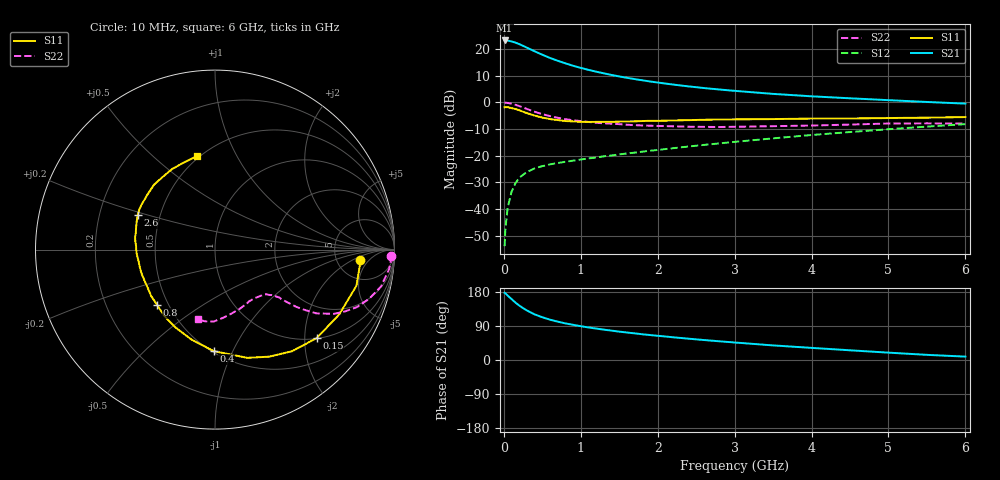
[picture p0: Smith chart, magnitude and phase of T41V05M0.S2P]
! Infineon Technologies  Discrete & RF Semiconductors
! BFR182T
! Si NPN RF Bipolar Junction Transistor in SC75
! VCE = 1 V  IC = 5 mA
! Common Emitter S-Parameters:  October  1999
# GHz  S  MA  R  50
!  f  S11  S21  S12  S22
! GHz  MAG  ANG  MAG  ANG  MAG  ANG  MAG  ANG
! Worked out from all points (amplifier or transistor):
!   36 points, 10 MHz to 6 GHz, reference 50 ohm
!   highest |S21| = 23.2 dB at 10 MHz (marker M1)
!   |S21| within 3 dB of that: start of sweep to 321.7 MHz
!   unconditionally stable (mu >= 1): 1.274 GHz to 4.316 GHz
!   at 250 MHz: K = 0.30, MSG = 24.2 dB, |S12| = -27.2 dB
!   at 1.4 GHz: K = 1.04, MAG = 13.8 dB, |S12| = -19.9 dB
!   at 6 GHz: K = 0.89, MSG = 3.9 dB, |S12| = -8.2 dB
!   S11 on the Smith chart (normalised r, x): 10 MHz: 8.54, -2.78; 150 MHz: 1.01, -2.29; 400 MHz: 0.51, -0.85; 800 MHz: 0.43, -0.34; 2.6 GHz: 0.37, +0.18; 6 GHz: 0.49, +0.70
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0.01  0.8087 -4.0  14.53 177.3  0.002 84.8  0.9805 -2.0
0.02  0.8136 -4.4  14.46 176.3  0.0042 92.8  0.9845 -2.6
0.05  0.8134 -14.3  14.46 170.0  0.0106 87.4  0.9762 -6.4
0.1  0.7809 -27.5  13.93 160.8  0.0209 77.8  0.9478 -12.5
0.15  0.7512 -41.0  13.24 151.6  0.0304 70.2  0.9016 -17.7
0.2  0.7107 -52.8  12.41 143.8  0.0382 65.7  0.8528 -22.1
0.25  0.6688 -63.1  11.51 136.9  0.0439 60.3  0.7997 -25.6
0.3  0.6293 -73.4  10.64 130.7  0.0493 58.3  0.7527 -28.4
0.4  0.5653 -90.8  9.101 120.4  0.0577 53.1  0.6666 -32.2
0.5  0.5179 -104.7  7.839 112.8  0.0636 50.7  0.6024 -33.9
0.6  0.4865 -116.9  6.826 106.4  0.0686 49.8  0.5527 -35.2
0.7  0.4657 -127.3  6.044 101.2  0.0727 49.3  0.5144 -35.8
0.8  0.4465 -136.2  5.409 96.6  0.0767 49.3  0.4848 -36.3
1.1  0.4292 -157.3  4.078 85.8  0.0887 51.1  0.4293 -37.5
1.4  0.4308 -171.6  3.27 77.5  0.1007 52.9  0.3979 -39.5
1.6  0.4393 -179.8  2.891 72.5  0.1099 54.2  0.3805 -40.8
2.2  0.4572 164.0  2.16 60.0  0.138 57.2  0.3558 -47.9
2.6  0.4713 155.9  1.86 52.7  0.1591 58.4  0.3471 -53.5
3.5  0.4858 140.5  1.443 38.5  0.2111 58.2  0.3576 -67.3
4.5  0.4986 126.1  1.193 25.6  0.2776 55.0  0.3832 -83.5
5.5  0.5164 109.0  1.018 13.6  0.351 49.9  0.4036 -97.7
6  0.53 100.8  0.948 8.9  0.3902 46.2  0.4005 -103.9
